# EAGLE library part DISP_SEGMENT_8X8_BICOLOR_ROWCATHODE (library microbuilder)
8x8 Bi-Color LED Segment Displays: Row = Cathode 1.2" Bi-Color 8x8 Matrix, 3.0mm Square LEDs - BL-M12A883XX
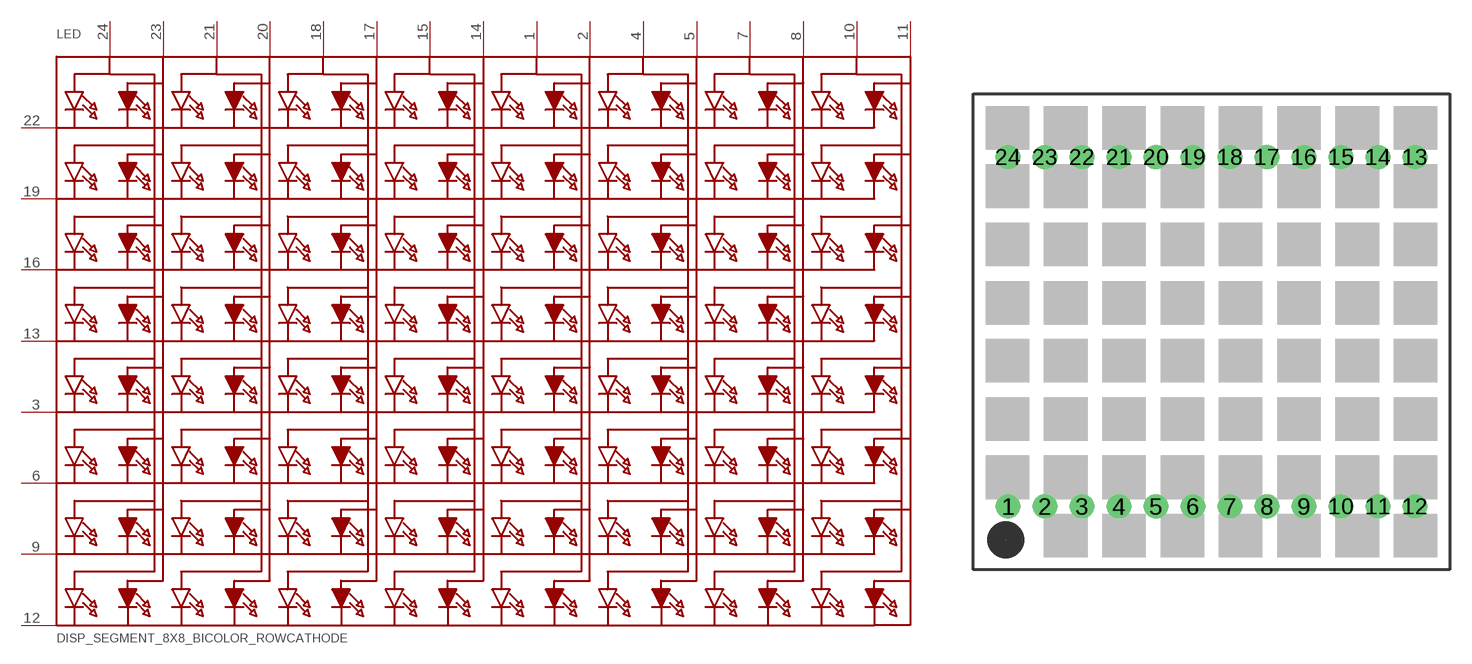
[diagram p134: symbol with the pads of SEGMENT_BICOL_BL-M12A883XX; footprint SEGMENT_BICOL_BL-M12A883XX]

Designator prefix LED

## DISP_SEGMENT_8X8_BICOLOR_ROWCATHODEMI2A883XX  [SEGMENT_BICOL_BL-M12A883XX]
1  A9
2  A10
3  K5
4  A11
5  A12
6  K6
7  A13
8  A14
9  K7
10  A15
11  A16
12  K8
13  K4
14  A8
15  A7
16  K3
17  A6
18  A5
19  K2
20  A4
21  A3
22  K1
23  A2
24  A1

## Footprint SEGMENT_BICOL_BL-M12A883XX (pad centres in mm)
Source: http://www.betlux.com/product/led_dot_matrix/BL-M12A883xx.PDF
drill 0.8 pad 1.676: 1 -13.97,-12; 2 -11.43,-12; 3 -8.89,-12; 4 -6.35,-12; 5 -3.81,-12; 6 -1.27,-12; 7 1.27,-12; 8 3.81,-12; 9 6.35,-12; 10 8.89,-12; 11 11.43,-12; 12 13.97,-12; 13 13.97,12; 14 11.43,12; 15 8.89,12; 16 6.35,12; 17 3.81,12; 18 1.27,12; 19 -1.27,12; 20 -3.81,12; 21 -6.35,12; 22 -8.89,12; 23 -11.43,12; 24 -13.97,12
